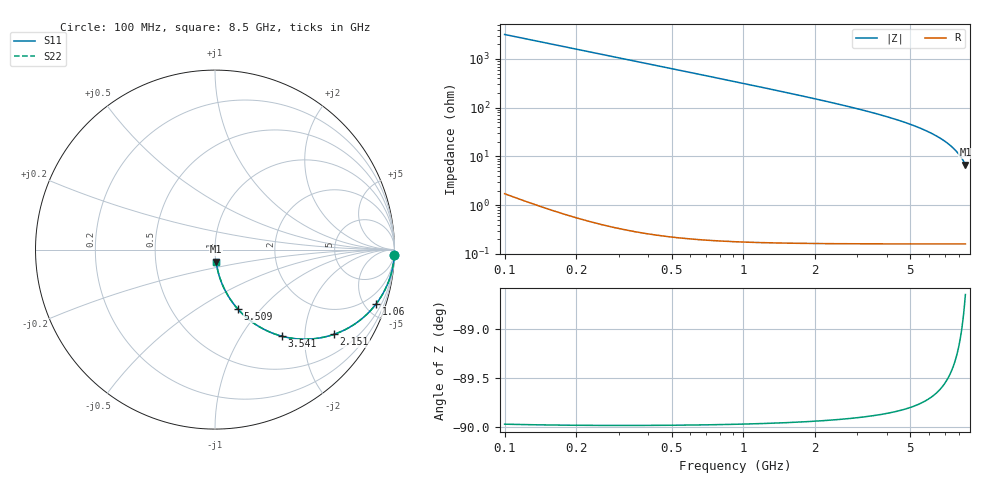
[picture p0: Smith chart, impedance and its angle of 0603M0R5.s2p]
! Created Wed Apr 18 11:55:49 2012
# hz S ma R 50
! 2 Port Network Data from SP1.SP block
! freq  magS11  angS11  magS21  angS21  magS12  angS12  magS22  angS22
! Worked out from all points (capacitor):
!   8401 points, 100 MHz to 8.5 GHz, reference 50 ohm
!   read as one part in series: C = 500 fF near 142 MHz
!   lowest |Z| = 6.81 ohm at 8.5 GHz (marker M1)
!   S11 on the Smith chart (normalised r, x): 100 MHz: 1, -64; 1.06 GHz: 1.00, -5.93; 2.151 GHz: 1.00, -2.80; 3.541 GHz: 1.00, -1.54; 5.509 GHz: 1.00, -0.76; 8.5 GHz: 1.00, -0.14
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1e8  0.9995 -1.8  0.0314 88.2  0.0314 88.2  0.9995 -1.8
1.24e8  0.9992 -2.2  0.03893 87.7  0.03893 87.7  0.9992 -2.2
1.85e8  0.9983 -3.3  0.05804 86.7  0.05804 86.7  0.9983 -3.3
2.44e8  0.997 -4.4  0.07648 85.6  0.07648 85.6  0.997 -4.4
3.27e8  0.9947 -5.9  0.1023 84.1  0.1023 84.1  0.9947 -5.9
4.27e8  0.991 -7.7  0.1332 82.3  0.1332 82.3  0.991 -7.7
5.51e8  0.9852 -9.9  0.1711 80.1  0.1711 80.1  0.9852 -9.9
6.97e8  0.9765 -12.4  0.215 77.6  0.215 77.6  0.9765 -12.4
8.66e8  0.9642 -15.3  0.2646 74.6  0.2646 74.6  0.9642 -15.3
1.06e9  0.9474 -18.6  0.3195 71.3  0.3195 71.3  0.9474 -18.6
1.5e9  0.9 -25.8  0.4352 64.2  0.4352 64.2  0.9 -25.8
2.151e9  0.8138 -35.5  0.5803 54.5  0.5803 54.5  0.8138 -35.5
2.9e9  0.7041 -45.1  0.7089 44.8  0.7089 44.8  0.7041 -45.1
3.541e9  0.6102 -52.3  0.791 37.6  0.791 37.6  0.6102 -52.3
4.3e9  0.5046 -59.5  0.862 30.3  0.862 30.3  0.5046 -59.5
5.509e9  0.3542 -69.0  0.9337 20.7  0.9337 20.7  0.3542 -69.0
5.7e9  0.3325 -70.3  0.9416 19.4  0.9416 19.4  0.3325 -70.3
6.457e9  0.2516 -75.1  0.9663 14.6  0.9663 14.6  0.2516 -75.1
7.1e9  0.1887 -78.6  0.9805 10.9  0.9805 10.9  0.1887 -78.6
7.889e9  0.1181 -82.4  0.9914 6.8  0.9914 6.8  0.1181 -82.4
8.192e9  0.09272 -83.7  0.9941 5.3  0.9941 5.3  0.09272 -83.7
8.5e9  0.0678 -84.8  0.9961 3.9  0.9961 3.9  0.0678 -84.8
